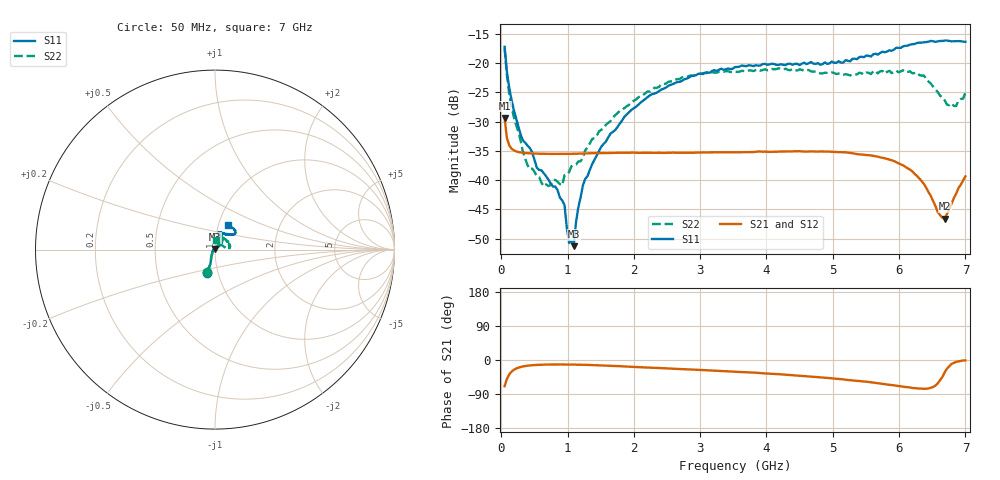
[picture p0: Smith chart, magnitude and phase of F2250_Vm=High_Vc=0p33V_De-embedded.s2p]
! Integrated Device Technology
! Corporate Headquarters
! 6024 Silver Creek Valley Road
! San Jose, CA 95138  USA
! Phone:  1-408-284-8200
! Toll Free:  1-800-223-1366
! Webpage:  http://www.idt.com/
! Timing and RF Division
! 515 Groton Road, Suite 102
! Westford, MA 01886-6024
! Device:  F2250
! Description: Voltage Variable RF Attenuator
! Frequency:  50.0 -  6000.00 MHz
! Package:  3x3 mm Thin QFN Plastic Package: 16 pin
! Ports:  2 RF, 3 DC
!  Pin  1  = GND
!  Pin  2  = NC
!  Pin  3  = RF1  = Port 1
!  Pin  4  = NC
!  Pin  5  = GND
!  Pin  6  = GND
!  Pin  7  = GND
!  Pin  8  = GND
!  Pin  9  = NC
!  Pin 10  = RF2  = Port 2
!  Pin 11  = NC
!  Pin 12  = GND
!  Pin 13  = GND
!  Pin 14  = VCNTRL
!  Pin 15  = VDD
!  Pin 16  = VMODE
! Vcntrl:  0.330 Volts
! Vmode:  +3.300 Volts
! Vdd:  +3.30  Volts
! Current:  1.255 mA
! Data:  The device was measured on a the F2250 evaluation board which has
!  individual transmission lines to the RF pins.  Data was collected
!  using a calibrated network analyzer.  The evaluation board was
!  de-embedded using a TRL calibration technique.
!  The reference plane is the edge of the package pin.
! Misc:  SN 10
!  Action Tracker AT0258
! Date Measured:  2014-11-26
! Date:  2015-10-15  MJV
! Note:
!  Integrated Device Technology supplies this data as a sample of measured
!  data at the package pin for this product.  Your particular data for this
!  product may vary.
!  Data was taken at 25 degrees C.
!  Integrated Device Technology reserves the right to change this data at anytime.
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# GHz S dB R 50
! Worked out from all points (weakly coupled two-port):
!   201 points, 50 MHz to 7 GHz, reference 50 ohm
!   highest |S21| = -29.35 dB at 50 MHz (marker M1); lowest = -46.6 dB at 6.687 GHz (marker M2)
!   lowest |S11| = -51.3 dB at 1.093 GHz (marker M3), VSWR 1.01, Z = 50 + j0.272 ohm
!   |S11| at or under -10 dB: start of sweep to end of sweep
!   |S22| runs from -41.0 to -17.5 dB; largest |S21 - S12| = 5.2e-05
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0.05  -17.18 -108.5  -29.35 -69.1  -29.35 -69.1  -17.49 -110.0
0.08475  -21.48 -107.4  -32.80 -49.8  -32.80 -49.8  -22.04 -107.7
0.189  -28.00 -120.0  -34.90 -26.0  -34.90 -26.0  -29.19 -121.3
0.29325  -32.27 -127.4  -35.27 -18.4  -35.26 -18.3  -33.34 -128.6
0.3975  -34.11 -142.2  -35.39 -15.0  -35.39 -15.0  -37.49 -154.0
0.64075  -38.81 -162.6  -35.49 -12.2  -35.49 -12.2  -41.05 157.5
0.91875  -43.45 156.0  -35.51 -11.8  -35.51 -11.8  -40.88 117.9
0.9535  -44.28 170.8  -35.51 -11.8  -35.51 -11.9  -39.16 115.5
1.023  -50.76 140.6  -35.50 -11.9  -35.50 -12.0  -38.60 97.8
1.0925  -51.29 88.6  -35.49 -12.1  -35.49 -12.1  -37.43 88.6
1.12725  -47.17 61.3  -35.47 -12.2  -35.48 -12.2  -37.33 81.7
1.2315  -40.85 40.7  -35.44 -12.6  -35.44 -12.6  -36.14 67.9
1.3705  -37.27 37.5  -35.38 -13.5  -35.39 -13.5  -32.96 60.5
1.6485  -32.02 41.2  -35.35 -15.3  -35.35 -15.3  -29.88 55.4
2.37825  -24.76 46.7  -35.32 -21.2  -35.31 -21.2  -24.06 51.6
3.525  -20.65 71.7  -35.24 -30.9  -35.24 -30.9  -21.44 71.8
4.7065  -20.06 72.0  -35.08 -44.2  -35.09 -44.2  -21.43 69.6
5.85325  -17.79 40.5  -36.49 -65.1  -36.50 -65.2  -21.29 22.2
6.3745  -16.40 40.9  -40.65 -76.0  -40.66 -76.1  -22.11 6.1
6.68725  -16.12 47.9  -46.61 -32.7  -46.60 -32.4  -26.33 27.5
6.861  -16.22 54.5  -42.29 -5.0  -42.25 -5.1  -27.32 57.6
7  -16.32 62.4  -39.35 -1.2  -39.33 -1.3  -25.04 84.6
